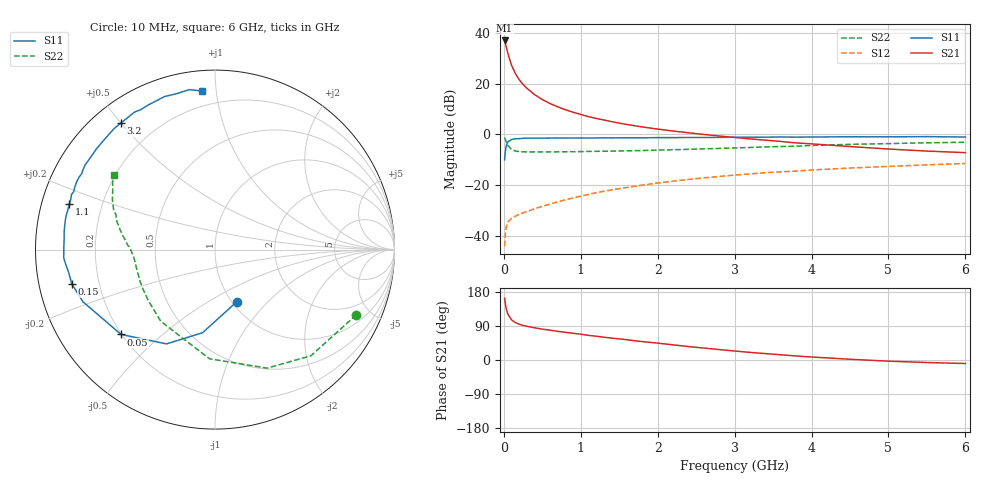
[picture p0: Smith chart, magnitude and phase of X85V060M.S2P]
! SIEMENS Small Signal Semiconductors
! BFP136W
! Si NPN RF Bipolar Junction Transistor in SOT343
! VCE = 5 V  IC = 60 mA
! Common Emitter S-Parameters:  September  1994
# GHz  S  MA  R  50
!  f  S11  S21  S12  S22
! GHz  MAG  ANG  MAG  ANG  MAG  ANG  MAG  ANG
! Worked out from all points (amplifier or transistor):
!   40 points, 10 MHz to 6 GHz, reference 50 ohm
!   highest |S21| = 37.1 dB at 10 MHz (marker M1)
!   |S21| within 3 dB of that: start of sweep to 35.65 MHz
!   unconditionally stable (mu >= 1): 676.8 MHz to 2.915 GHz
!   at 200 MHz: K = 0.58, MSG = 26.6 dB, |S12| = -31.5 dB
!   at 1.5 GHz: K = 1.10, MAG = 11.0 dB, |S12| = -21.4 dB
!   at 6 GHz: K = 0.96, MSG = 2.1 dB, |S12| = -11.5 dB
!   S11 on the Smith chart (normalised r, x): 10 MHz: 1.06, -0.68; 50 MHz: 0.20, -0.37; 150 MHz: 0.10, -0.12; 1.1 GHz: 0.08, +0.15; 3.2 GHz: 0.08, +0.50; 6 GHz: 0.11, +0.91
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0.01  0.3144 -67.1  71.59 162.7  0.0062 72.2  0.8669 -24.8
0.02  0.4682 -98.5  63.26 147.9  0.0111 61.5  0.7974 -47.9
0.03  0.5908 -117.2  55.2 136.5  0.0146 52.1  0.7214 -66.3
0.05  0.7052 -137.9  40.81 121.8  0.0183 40.8  0.609 -92.9
0.1  0.7914 -158.5  23.2 105.9  0.0221 33.8  0.5008 -127.1
0.15  0.8203 -166.5  15.91 98.7  0.0243 34.8  0.4677 -142.7
0.2  0.8251 -171.1  12 94.4  0.0265 36.1  0.4574 -151.4
0.25  0.8362 -174.5  9.679 91.3  0.0282 37.3  0.4537 -156.9
0.3  0.8442 -176.9  8.108 89.0  0.0298 40.2  0.4501 -160.7
0.4  0.8423 179.1  6.106 84.9  0.034 43.7  0.4495 -165.7
0.5  0.8426 175.9  4.87 81.5  0.0378 47.1  0.4498 -169.0
0.6  0.8456 173.7  4.065 78.7  0.0422 49.7  0.4509 -171.1
0.7  0.848 171.1  3.505 75.6  0.0466 52.3  0.4522 -172.5
0.9  0.8508 167.2  2.74 70.5  0.0556 54.6  0.4551 -175.2
1.1  0.8504 162.7  2.241 64.9  0.0652 55.9  0.4602 -176.9
1.5  0.8552 156.0  1.667 55.7  0.0848 57.0  0.4698 -179.9
1.8  0.8547 150.4  1.403 48.6  0.0995 55.9  0.4794 177.9
2.2  0.8631 143.5  1.164 40.0  0.1192 53.6  0.4964 175.0
3.2  0.8793 126.6  0.814 20.1  0.1658 45.5  0.5511 166.3
4.5  0.8979 108.3  0.575 2.0  0.2163 34.0  0.6348 154.2
5.5  0.9027 99.1  0.468 -6.6  0.25 26.2  0.6817 146.8
6  0.8868 94.8  0.436 -9.3  0.2667 21.9  0.6992 143.6
